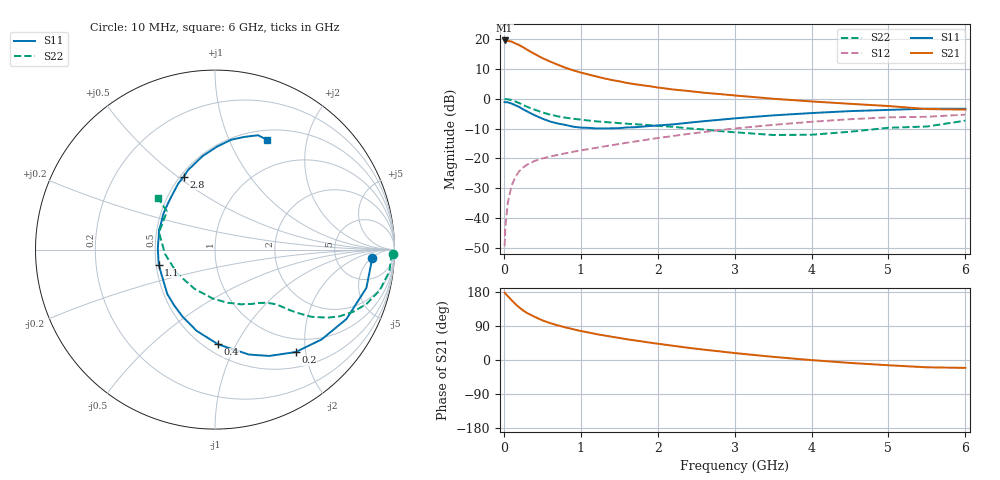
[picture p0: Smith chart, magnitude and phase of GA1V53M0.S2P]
! Infineon Technologies  Discrete & RF Semiconductors
! BF775
! Si NPN RF Bipolar Junction Transistor in SOT23
! VCE = 1.5 V  IC = 3 mA
! Common Emitter S-Parameters:  May  1996
# GHz  S  MA  R  50
!  f  S11  S21  S12  S22
! GHz  MAG  ANG  MAG  ANG  MAG  ANG  MAG  ANG
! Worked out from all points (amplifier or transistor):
!   36 points, 10 MHz to 6 GHz, reference 50 ohm
!   highest |S21| = 19.5 dB at 10 MHz (marker M1)
!   |S21| within 3 dB of that: start of sweep to 296.2 MHz
!   unconditionally stable (mu >= 1): 938.8 MHz to 4.465 GHz; 5.01 GHz to end of sweep
!   at 250 MHz: K = 0.37, MSG = 20.1 dB, |S12| = -23.0 dB
!   at 1.4 GHz: K = 1.15, MAG = 8.6 dB, |S12| = -15.6 dB
!   at 6 GHz: K = 1.02, MAG = 0.0 dB, |S12| = -5.4 dB
!   S11 on the Smith chart (normalised r, x): 10 MHz: 13, -5; 200 MHz: 0.75, -1.81; 400 MHz: 0.58, -0.85; 1.1 GHz: 0.52, -0.10; 2.8 GHz: 0.52, +0.53; 6 GHz: 0.62, +1.40
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0.01  0.8763 -2.9  9.428 178.0  0.0034 87.7  0.9942 -1.4
0.02  0.8727 -5.8  9.347 175.3  0.0072 85.6  0.9825 -2.8
0.05  0.87 -14.2  9.252 168.8  0.0178 81.8  0.9792 -7.1
0.1  0.8284 -27.8  9.031 158.1  0.0349 75.2  0.9461 -13.8
0.15  0.7769 -40.1  8.402 147.5  0.049 68.0  0.8964 -19.8
0.2  0.7265 -51.8  7.865 138.8  0.0612 63.2  0.8434 -24.3
0.25  0.665 -63.0  7.274 130.8  0.0705 58.3  0.7854 -28.3
0.3  0.6143 -72.1  6.627 124.3  0.0783 55.3  0.7339 -31.1
0.4  0.5284 -88.1  5.604 114.0  0.0908 50.8  0.6545 -34.9
0.5  0.4639 -102.8  4.787 104.7  0.0997 48.5  0.5896 -37.1
0.6  0.4153 -115.8  4.194 97.5  0.1073 47.2  0.5417 -38.8
0.7  0.3845 -126.5  3.705 91.4  0.1146 46.7  0.5074 -39.9
0.9  0.3401 -146.4  2.984 81.2  0.1294 46.4  0.4623 -41.7
1.1  0.3248 -165.0  2.538 72.6  0.1432 46.9  0.4311 -44.0
1.3  0.3185 179.8  2.195 65.0  0.1587 47.4  0.4076 -46.5
1.6  0.3302 161.0  1.835 54.7  0.1829 47.5  0.3812 -51.3
2.2  0.3716 133.7  1.425 37.5  0.2374 45.6  0.338 -64.5
2.8  0.4427 113.2  1.196 22.9  0.2973 41.1  0.2871 -83.6
3.5  0.5254 97.6  0.998 8.3  0.3644 33.5  0.2467 -117.3
4.5  0.6193 81.5  0.821 -7.7  0.4534 20.6  0.2795 -175.0
5.5  0.6806 69.4  0.671 -19.3  0.498 6.0  0.342 141.5
6  0.6768 64.4  0.656 -20.8  0.5397 2.0  0.4283 137.9
